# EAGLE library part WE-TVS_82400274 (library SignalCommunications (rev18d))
TVS Diode High Speed Series Characteristics Low clamping voltage Sturdy design Very low capacitance Flow Thru Design for a simple layout Rail to Rail protection Epoxy flame resistant UL94 V-0 RoHS, REACH and free of halogens Applications Very fast data lines USB 2.0 Ethernet PoE VGA Sim Cards Keypads ESD protection in accordance with EN 61000-4-2, – 8 kV contact discharge – 15 kV air discharge Details see: http://katalog.we-online.de/pbs/datasheet/82400274.pdf Updated by Dan Xu 2014-07-11 2014 (C) Wurth Elektronik
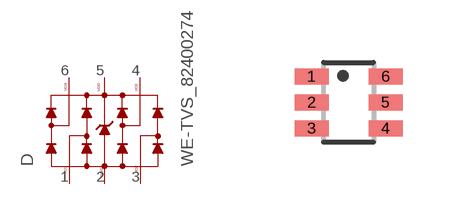
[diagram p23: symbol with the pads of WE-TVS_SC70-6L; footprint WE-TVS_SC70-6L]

Designator prefix D

## WE-TVS_82400274  [WE-TVS_SC70-6L]
1  1
2  GND  pwr
3  3
4  4
5  VDD  pwr
6  6

## Footprint WE-TVS_SC70-6L (pad centres in mm)
TVS Diode Array WE-TVS
smd 0.85 x 0.4: 1 -0.925,0.65; 2 -0.925,0; 3 -0.925,-0.65; 4 0.925,-0.65; 5 0.925,0; 6 0.925,0.65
